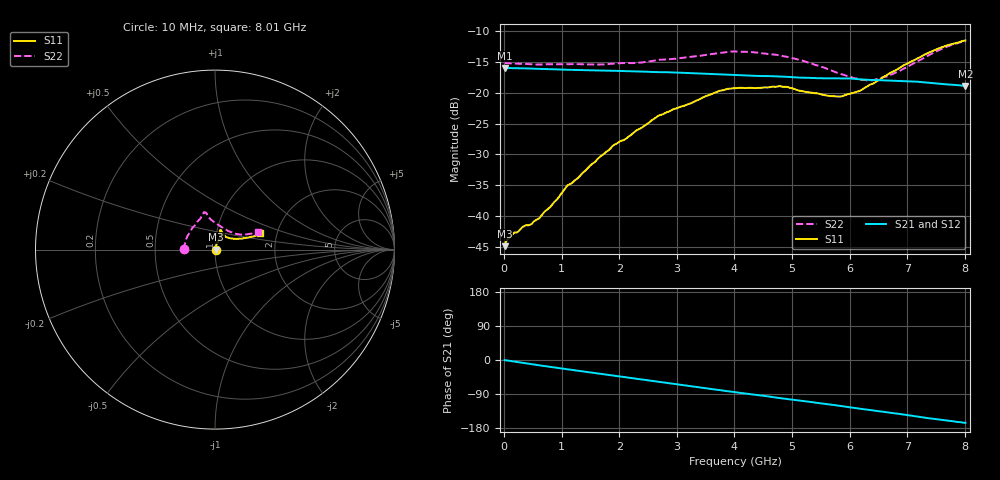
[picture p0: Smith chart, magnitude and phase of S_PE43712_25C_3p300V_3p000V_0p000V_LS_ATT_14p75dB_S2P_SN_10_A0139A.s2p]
! DEVICE ID: PE43712
! File Path: z:\PE43713\PE43713_CHAR_NOM_04292014\AMB\3p300\LS_ATT_14p75dB\PE43713_AMB_3p300V_3p000V_0p000V_LS_ATT_14p75dB_S2P_SN_10_A0139A.s2p
! Serial: 10
! Lot: A0139A
! Temp: 25C
! VDD: 3.300
! VSS: 0.000
! Control_Hi: 3.000
! Control_Lo: 0.000
! Attenuation Step: 14.75dB
! Port 1: RF1
! Port 2: RF2
! ThroughPath:1-2
! IDD: 0.0001471956
! ISS: -1.37e-007
#  Hz  S  RI  R  50
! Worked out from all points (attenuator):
!   801 points, 10 MHz to 8.01 GHz, reference 50 ohm
!   highest |S21| = -15.96 dB at 10 MHz (marker M1); lowest = -18.9 dB at 8.01 GHz (marker M2)
!   lowest |S11| = -44.9 dB at 10 MHz (marker M3), VSWR 1.01, Z = 50.6 + j0.0425 ohm
!   |S11| at or under -10 dB: start of sweep to end of sweep
!   |S22| runs from -18.0 to -11.7 dB; largest |S21 - S12| = 0.00059
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1e7  0.00567 0.00042  0.1593 -0.000802  0.1594 -0.000767  -0.1752 0.00111
1.6e8  0.0068 0.00231  0.1584 -0.0106  0.1585 -0.0106  -0.1729 0.0117
6.1e8  0.00627 0.00723  0.1521 -0.0379  0.1521 -0.0379  -0.1657 0.0379
9.1e8  0.00527 0.0124  0.1454 -0.0544  0.1455 -0.0544  -0.1616 0.0553
1.09e9  0.00525 0.0166  0.1405 -0.0635  0.1406 -0.0635  -0.1572 0.0665
1.35e9  0.00612 0.0212  0.1331 -0.0759  0.1331 -0.0759  -0.1506 0.08
1.9e9  0.0116 0.0357  0.1138 -0.0994  0.1138 -0.0994  -0.1311 0.1128
2.11e9  0.014 0.0398  0.1053 -0.1073  0.1053 -0.1073  -0.1241 0.1227
2.68e9  0.0254 0.0601  0.0795 -0.1241  0.0794 -0.1242  -0.0957 0.1592
3.72e9  0.0317 0.098  0.0271 -0.139  0.027 -0.139  -0.065 0.2001
4.01e9  0.0316 0.1047  0.0125 -0.1395  0.0125 -0.1394  -0.0624 0.2077
4.79e9  0.0321 0.1086  -0.0246 -0.1335  -0.0246 -0.1337  -0.0448 0.1963
5.35e9  0.0432 0.0902  -0.0481 -0.1232  -0.0481 -0.1231  -0.0264 0.1705
5.64e9  0.0535 0.0778  -0.0592 -0.1173  -0.0592 -0.1173  -0.00601 0.1544
5.87e9  0.0634 0.0692  -0.069 -0.1115  -0.0689 -0.1115  0.0138 0.1407
6.16e9  0.0814 0.0634  -0.0798 -0.1013  -0.0796 -0.1015  0.0436 0.1213
6.3e9  0.094 0.0614  -0.0836 -0.0967  -0.0834 -0.0967  0.0602 0.1114
6.42e9  0.1033 0.0606  -0.0869 -0.0928  -0.0867 -0.0928  0.0737 0.1036
6.68e9  0.1298 0.0604  -0.0943 -0.0834  -0.094 -0.0834  0.1046 0.0907
7.37e9  0.1996 0.071  -0.1082 -0.0538  -0.1081 -0.0538  0.1822 0.0861
7.72e9  0.232 0.0796  -0.1102 -0.0391  -0.1101 -0.0392  0.222 0.093
8.01e9  0.2508 0.0903  -0.1103 -0.0279  -0.1102 -0.0282  0.2422 0.0965
